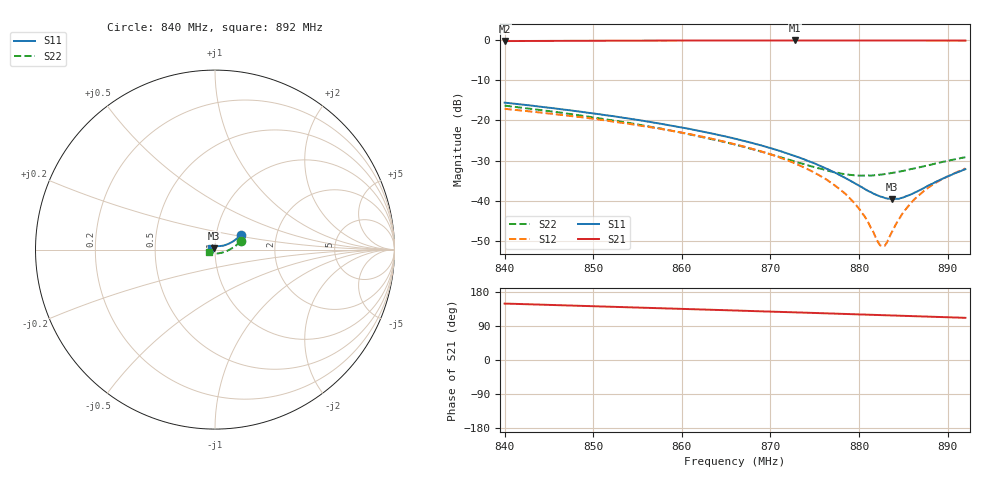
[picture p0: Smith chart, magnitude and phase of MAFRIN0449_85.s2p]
!Part Number:  MAFRIN0449
!Name:  MariaCraven
!Comments:  1
!Thu 30/Sep/2004  2:08:29 PM
!Temperature:  85
# MHZ  S  DB  R  50
!Freq  S11(dB)  S11(ang)  S21(dB)  S21(ang)  S12(dB)  S12(ang)  S22(dB)  S22(ang)
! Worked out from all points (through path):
!   201 points, 840 MHz to 892 MHz, reference 50 ohm
!   highest |S21| = -0.24 dB at 872.8 MHz (marker M1); lowest = -0.4 dB at 840 MHz (marker M2)
!   lowest |S11| = -39.5 dB at 883.7 MHz (marker M3), VSWR 1.02, Z = 49.3 + j0.767 ohm
!   |S11| at or under -10 dB: start of sweep to end of sweep
!   |S22| runs from -33.7 to -16.4 dB; largest |S21 - S12| = 0.98
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840  -15.65 29.6  -0.39 148.8  -17.18 101.1  -16.38 18.1
848.84  -17.97 25.8  -0.32 142.8  -19.32 93.8  -18.92 9.6
857.42  -20.80 23.4  -0.27 136.7  -22.08 87.1  -21.99 -0.9
866  -24.58 24.2  -0.25 130.6  -25.96 81.2  -26.04 -17.0
869.38  -26.52 27.0  -0.24 128.1  -28.01 79.4  -28.05 -27.2
872.76  -28.84 33.3  -0.24 125.8  -30.69 78.9  -30.23 -42.1
874.84  -30.57 41.4  -0.24 124.2  -32.84 79.7  -31.54 -54.5
877.44  -33.16 60.6  -0.24 122.2  -36.42 84.7  -32.99 -74.3
878.48  -34.35 71.7  -0.24 121.5  -38.30 91.6  -33.40 -83.2
879.52  -35.62 85.9  -0.24 120.7  -40.62 107.7  -33.66 -91.8
880.82  -37.28 104.0  -0.24 119.7  -44.47 164.7  -33.70 -102.3
882.12  -38.66 119.2  -0.25 118.9  -50.15 -148.4  -33.58 -112.2
882.38  -38.89 121.8  -0.26 118.6  -51.02 -145.4  -33.49 -113.9
882.9  -39.26 126.4  -0.25 118.2  -51.12 -139.5  -33.35 -117.4
883.42  -39.45 130.3  -0.25 117.8  -48.97 -135.7  -33.16 -121.0
883.68  -39.54 132.5  -0.25 117.6  -47.82 -134.5  -33.09 -122.4
884.2  -39.47 135.6  -0.25 117.3  -45.61 -132.3  -32.87 -125.6
884.98  -39.16 139.7  -0.26 116.7  -42.86 -130.4  -32.56 -129.9
885.76  -38.48 142.9  -0.26 116.1  -40.74 -128.9  -32.15 -133.6
886.8  -37.39 146.2  -0.26 115.3  -38.49 -128.3  -31.68 -138.2
888.62  -35.32 150.6  -0.26 113.8  -35.55 -127.4  -30.74 -145.2
892  -32.14 154.4  -0.27 111.3  -31.97 -127.9  -29.16 -155.3
